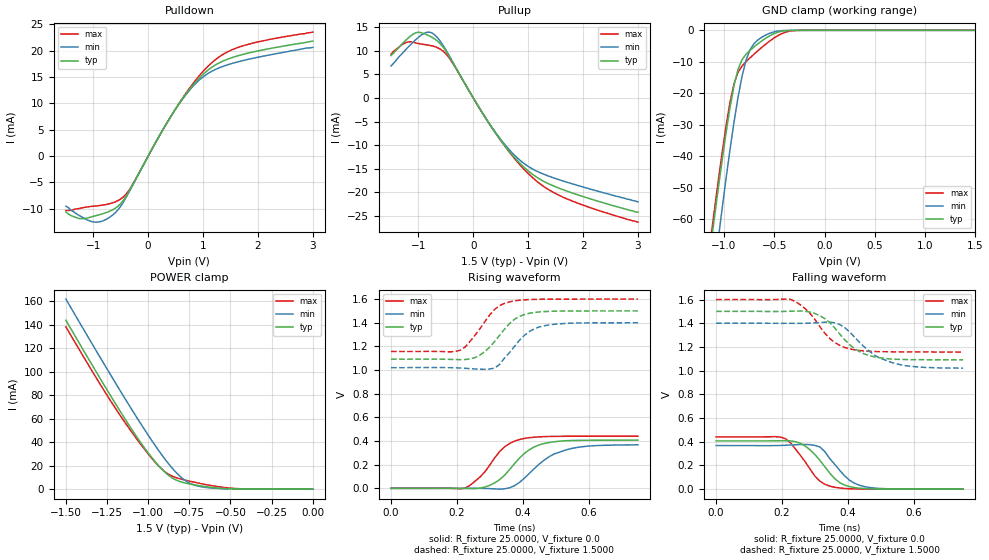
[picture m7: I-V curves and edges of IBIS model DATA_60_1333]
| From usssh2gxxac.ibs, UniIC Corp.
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|   Model DATA_60_1333
[Model]  DATA_60_1333
Model_type I/O
Polarity   Non-Inverting
Enable   Active-High
Vinl =   0.60000000V
Vinh =   0.90000000V
Vmeas =   0.750000000V
Rref =   25.00000000
Vref =   0.75000000V
C_comp   1.6160pF   1.5990pF   1.6430pF
[Temperature Range]   25.0000   95.0000   0.0
[Voltage Range]   1.5000V   1.4000V   1.6000V
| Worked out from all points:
|   slope of the pulldown table from 0 to 0.225 V, typ, clamps not added: 53.4 ohm
|   slope of the pullup table from 0 to 0.225 V, typ, clamps not added: 52.6 ohm
|   GND clamp passes 1 mA (typ) near -0.50 V on its own axis
|   POWER clamp passes 1 mA (typ) near -0.58 V on its own axis
|   rising waveform, R_fixture 25.0000, V_fixture 0.0: 20-80 % time 86.5ps typ, 99.4ps min, 79ps max; typ from 0 V to 0.407 V
|   rising waveform, R_fixture 25.0000, V_fixture 1.5000: 20-80 % time 78.8ps typ, 76.2ps min, 73.4ps max; typ from 1.09 V to 1.5 V
|   falling waveform, R_fixture 25.0000, V_fixture 0.0: 20-80 % time 75.8ps typ, 70.4ps min, 70.8ps max; typ from 0.407 V to 0 V
|   falling waveform, R_fixture 25.0000, V_fixture 1.5000: 20-80 % time 88.4ps typ, 99.9ps min, 81.8ps max; typ from 1.5 V to 1.09 V
[Pulldown]
|Voltage   I(typ)   I(min)   I(max)
-1.5V     -10.6mA    -9.5mA     -10.3mA
-1.25V    -11.86mA   -11.3mA    -9.93mA
-1V       -11.42mA   -12.48mA   -9.5mA
-800mV    -10.84mA   -12.17mA   -9.25mA
-600mV    -9.882mA   -10.74mA   -8.682mA
-350mV    -6.704mA   -6.838mA   -6.505mA
200mV     3.763mA    3.796mA    3.76mA
550mV     9.696mA    9.684mA    9.781mA
850mV     13.86mA    13.59mA    14.19mA
1.15V     16.76mA    16.02mA    17.61mA
1.75V     19.33mA    18.16mA    20.97mA
3V        21.8mA     20.6mA     23.5mA
[Pullup]
|Voltage   I(typ)   I(min)   I(max)
-1.5V     9mA        6.8mA      9.3mA
-1.25V    12.03mA    10mA       11.63mA
-1.05V    13.82mA    12.36mA    11.68mA
-900mV    13.65mA    13.69mA    11.34mA
-750mV    12.84mA    13.77mA    11.04mA
-600mV    11.47mA    12.01mA    10.35mA
-450mV    9.041mA    9.198mA    8.665mA
300mV     -5.62mA    -5.548mA   -5.6mA
850mV     -13.84mA   -13.18mA   -14.16mA
1.2V      -17.1mA    -15.73mA   -18.03mA
1.55V     -19.04mA   -17.25mA   -20.54mA
3V        -24.2mA    -22mA      -26.3mA
[GND_clamp]
|Voltage   I(typ)   I(min)   I(max)
-1.5V     -169mA     -189.1mA   -163.8mA
-1.14V    -70.71mA   -88.3mA    -68.32mA
-1.1V     -60.74mA   -77.66mA   -58.33mA
-1.06V    -51.03mA   -67.22mA   -48.61mA
-1.02V    -41.65mA   -57.06mA   -39.27mA
-940mV    -24.55mA   -37.9mA    -22.88mA
-860mV    -12.39mA   -21.26mA   -13.32mA
-780mV    -7.577mA   -9.433mA   -9.942mA
-740mV    -6.329mA   -6.125mA   -8.71mA
-620mV    -3.273mA   -2.113mA   -5.305mA
-300mV    -11.81uA   -4.878uA   -91.71uA
1.5V      4.577nA    23.6nA     33.33nA
[POWER_clamp]
|Voltage   I(typ)   I(min)   I(max)
-1.5V     143.7mA    161.7mA    138.1mA
-1.22V    77.56mA    95.29mA    73.32mA
-1.12V    55.19mA    72.34mA    52.54mA
-1.02V    34.59mA    50.23mA    33.56mA
-960mV    23.77mA    37.63mA    23.28mA
-900mV    14.66mA    25.9mA     15mA
-840mV    8.415mA    15.63mA    10.28mA
-780mV    5.408mA    7.848mA    7.861mA
-700mV    3.206mA    2.693mA    5.332mA
-600mV    1.29mA     794.5uA    2.681mA
-420mV    69.47uA    44.47uA    238.7uA
0V        4.577nA    6.249nA    39.08nA
[Ramp]
| variable   typ   min   max
dV/dt_r  0.2442/86.5366p   0.2207/98.3857p   0.2647/78.9981p
dV/dt_f  0.2448/88.3671p   0.2280/97.6364p   0.2658/81.8205p
R_load = 25.0000
[Rising Waveform]
R_fixture= 25.0000
V_fixture= 0.0
V_fixture_min= 0.0
V_fixture_max= 0.0
|time   V(typ)   V(min)   V(max)
0s        0V         0V         0V
225ps     -805.3uV   615uV      1.139mV
270ps     1.751mV    122.5uV    95.42mV
315ps     46.46mV    -4.577mV   258.4mV
360ps     157.9mV    4.509mV    378.8mV
405ps     295.1mV    85.55mV    422mV
480ps     387.4mV    267mV      438.4mV
530ps     402.5mV    323.8mV    440.3mV
605ps     406.3mV    358.3mV    441.1mV
750ps     407mV      367.8mV    441.2mV
[Rising Waveform]
R_fixture= 25.0000
V_fixture= 1.5000
V_fixture_min= 1.4000
V_fixture_max= 1.6000
|time   V(typ)   V(min)   V(max)
0s        1.092V     1.02V      1.157V
210ps     1.088V     1.017V     1.167V
225ps     1.089V     1.015V     1.194V
270ps     1.126V     1.007V     1.349V
315ps     1.242V     1.017V     1.513V
345ps     1.346V     1.102V     1.564V
375ps     1.429V     1.2V       1.585V
420ps     1.48V      1.325V     1.596V
465ps     1.494V     1.374V     1.599V
750ps     1.5V       1.4V       1.6V
[Falling Waveform]
R_fixture= 25.0000
V_fixture= 0.0
V_fixture_min= 0.0
V_fixture_max= 0.0
|time   V(typ)   V(min)   V(max)
0s        407mV      367.9mV    441.2mV
180ps     408.1mV    367.9mV    443mV
210ps     408.9mV    370.3mV    426.7mV
225ps     407.1mV    372.3mV    394mV
270ps     365mV      377.3mV    232.5mV
315ps     242.9mV    355.8mV    67.61mV
360ps     89.18mV    210mV      16.03mV
405ps     21.56mV    75.55mV    3.728mV
450ps     5.146mV    21.72mV    873.4uV
750ps     0V         0V         0V
[Falling Waveform]
R_fixture= 25.0000
V_fixture= 1.5000
V_fixture_min= 1.4000
V_fixture_max= 1.6000
|time   V(typ)   V(min)   V(max)
0s        1.5V       1.4V       1.6V
225ps     1.501V     1.399V     1.602V
270ps     1.501V     1.4V       1.524V
300ps     1.482V     1.403V     1.431V
360ps     1.361V     1.404V     1.238V
390ps     1.262V     1.364V     1.196V
435ps     1.161V     1.24V      1.17V
480ps     1.117V     1.133V     1.162V
530ps     1.098V     1.072V     1.159V
750ps     1.092V     1.021V     1.157V
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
